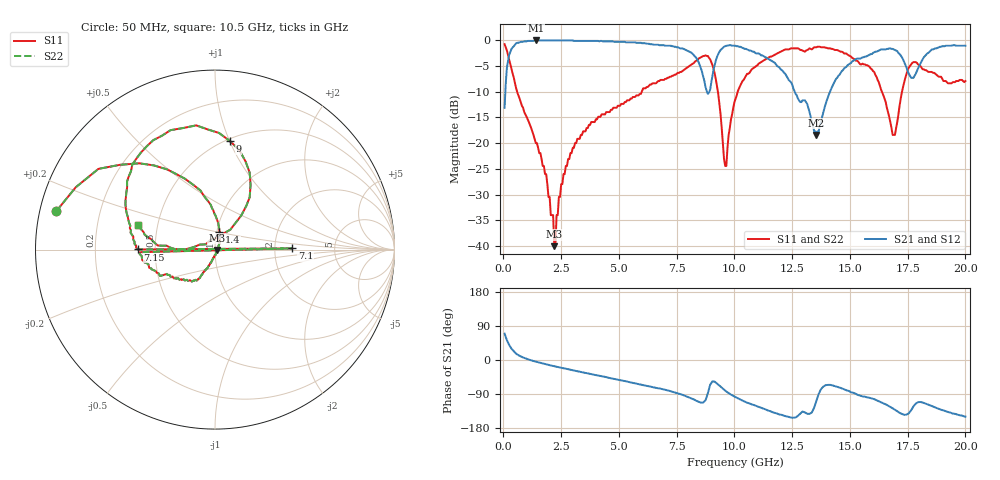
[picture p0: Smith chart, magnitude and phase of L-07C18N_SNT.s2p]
#	mhz	s	ma	r	50
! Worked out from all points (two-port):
!   400 points, 50 MHz to 20 GHz, reference 50 ohm
!   highest |S21| = -0.09 dB at 1.4 GHz (marker M1); lowest = -18.4 dB at 13.55 GHz (marker M2)
!   |S21| within 3 dB of the highest: 239.9 MHz to 8.273 GHz (8.033 GHz wide, 189 % of centre); 9.264 GHz to 11.25 GHz (1.982 GHz wide, 19.3 % of centre)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
!   lowest |S11| = -40.0 dB at 2.2 GHz (marker M3), VSWR 1.02, Z = 51 - j0.283 ohm
!   |S11| at or under -10 dB: 589.2 MHz to 5.991 GHz (5.402 GHz wide, 164 % of centre); 9.283 GHz to 10.14 GHz (861.1 MHz wide, 8.86 % of centre); 16.38 GHz to 17.26 GHz (874.1 MHz wide, 5.2 % of centre)
!   |S22| runs from -40.0 to -0.8 dB; largest |S21 - S12| = 0
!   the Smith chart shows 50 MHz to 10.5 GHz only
!   S11 on the Smith chart (normalised r, x): 50 MHz: 0.05, +0.12; 1.4 GHz: 1.03, +0.20; 7.1 GHz: 2.51, +0.04; 7.15 GHz: 0.40, +0.00; 9 GHz: 0.52, +1.00; 10.5 GHz: 0.39, +0.13
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50  0.91 166.4  0.22 69.4  0.22 69.4  0.91 166.4
550  0.34 103.9  0.93 16.4  0.93 16.4  0.34 103.9
1400  0.1 75.7  0.99 -4.3  0.99 -4.3  0.1 75.7
2200  0.01 -16.1  0.99 -16.4  0.99 -16.4  0.01 -16.1
2600  0.05 -100.6  0.99 -21.8  0.99 -21.8  0.05 -100.6
3400  0.12 -114.5  0.98 -32.2  0.98 -32.2  0.12 -114.5
6700  0.4 -169.8  0.9 -74.5  0.9 -74.5  0.4 -169.8
7050  0.42 -178.0  0.88 -79.5  0.88 -79.5  0.42 -178.0
7100  0.43 0.9  0.88 -80.1  0.88 -80.1  0.43 0.9
7150  0.43 179.9  0.88 -80.8  0.88 -80.8  0.43 179.9
8450  0.66 134.3  0.61 -110.2  0.61 -110.2  0.66 134.3
9000  0.61 82.1  0.39 -60.7  0.39 -60.7  0.61 82.1
9600  0.06 111.9  0.87 -80.7  0.87 -80.7  0.06 111.9
10050  0.27 175.4  0.88 -98.3  0.88 -98.3  0.27 175.4
10500  0.45 162.6  0.82 -111.3  0.82 -111.3  0.45 162.6
13350  0.81 75.7  0.16 -138.6  0.16 -138.6  0.81 75.7
13550  0.85 64.7  0.12 -107.4  0.12 -107.4  0.85 64.7
14650  0.77 13.2  0.5 -74.8  0.5 -74.8  0.77 13.2
16700  0.18 -13.5  0.83 -121.9  0.83 -121.9  0.18 -13.5
17550  0.54 41.5  0.47 -140.6  0.47 -140.6  0.54 41.5
18550  0.49 -22.2  0.81 -121.5  0.81 -121.5  0.49 -22.2
20000  0.4 -68.0  0.88 -149.4  0.88 -149.4  0.4 -68.0
